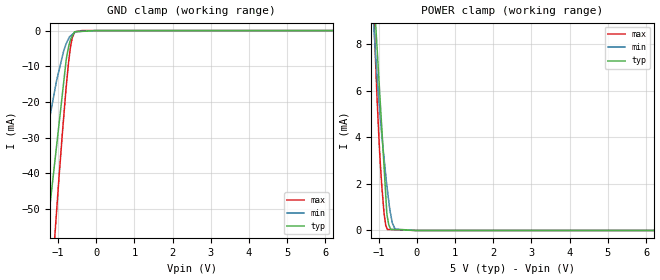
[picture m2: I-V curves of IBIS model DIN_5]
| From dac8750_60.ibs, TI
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[Model] DIN_5   |5V digital input
Model_type   Input
Vinl = 0.8
Vinh = 2
|   typ   min   max
|   (nom PVT)   (Fast PVT)   (slow PVT)
C_comp   1.959E-12   1.637E-12   2.239E-12
| Where   nom PVT is  Nominal Process, 5.0V, 36C
|   Fast PVT is Strong Process, 5.5V, -40C
|   Slow PVT is Weak Process, 4.5V, 134C
|C_comp - from L-C Tank method, L = 1nH, peak frequency
[Voltage Range]   5   4.5   5.5
|Operating Temperature   27   125   -40
|Junction Temperature
[Temperature Range]   36   134   -40
[Power Clamp Reference]   5   4.5   5.5
[GND Clamp Reference]   0   0   0
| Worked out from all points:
|   GND clamp passes 1 mA (typ) near -0.60 V on its own axis
|   POWER clamp passes 1 mA (typ) near -0.79 V on its own axis
[GND Clamp]
|   Voltage   I(typ)   I(min)   I(max)
-5V       -570.1mA   -391mA     -702.1mA
-1.681V   -106.1mA   -57.85mA   -154.2mA
-1.39V    -69.68mA   -35.78mA   -106.8mA
-1.249V   -52.82mA   -26.39mA   -83.76mA
-1.107V   -39.18mA   -18.15mA   -61.43mA
-1.036V   -32.4mA    -14.06mA   -50.79mA
-886.5mV  -18.05mA   -7.364mA   -29.13mA
-784.3mV  -8.257mA   -3.666mA   -15.92mA
-674.1mV  -2.59mA    -1.532mA   -4.816mA
-619.9mV  -1.434mA   -1.057mA   -1.823mA
-563.7mV  -338.8uA   -562.1uA   -481.1uA
9.985V    0A         0A         0A
[POWER Clamp]
|   Voltage   I(typ)   I(min)   I(max)
-5V       172.5mA    139.1mA    212.4mA
-1.149V   10.89mA    9.379mA    10.41mA
-1.09V    9.254mA    7.857mA    7.766mA
-1.066V   8.585mA    7.235mA    6.769mA
-984.6mV  6.326mA    5.44mA     3.776mA
-915.5mV  4.401mA    4.112mA    1.924mA
-848mV    2.522mA    2.972mA    631uA
-784.3mV  751.2uA    1.954mA    104.7uA
-770mV    583.3uA    1.761mA    42.55uA
-640.4mV  47.46uA    326.2uA    34.97uA
-567.8mV  42.18uA    61.14uA    30.73uA
9.985V    0A         0A         0A
